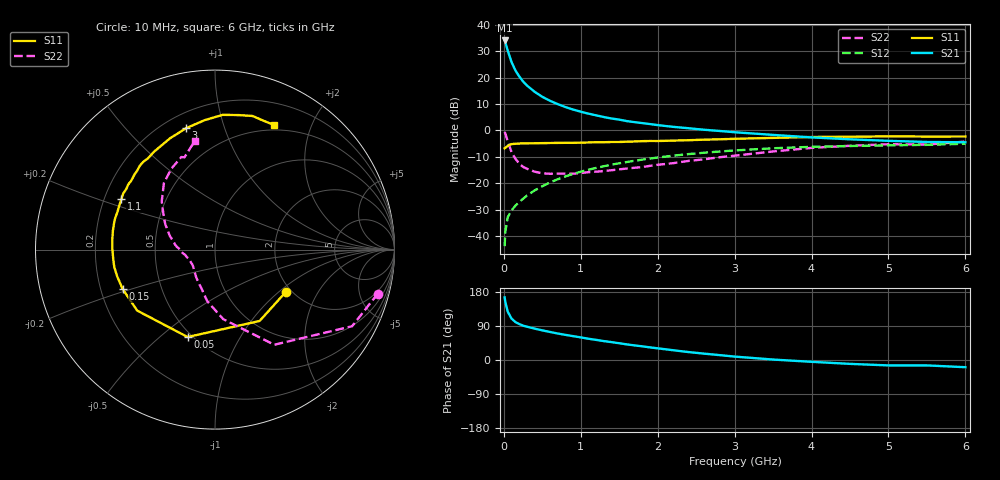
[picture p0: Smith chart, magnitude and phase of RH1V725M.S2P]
! SIEMENS Small Signal Semiconductors
! BFR106
! Si NPN RF Bipolar Junction Transistor in SOT23
! VCE = 1.75 V  IC = 25 mA
! Common Emitter S-Parameters:  August  1996
# GHz  S  MA  R  50
!  f  S11  S21  S12  S22
! GHz  MAG  ANG  MAG  ANG  MAG  ANG  MAG  ANG
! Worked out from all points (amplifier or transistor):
!   36 points, 10 MHz to 6 GHz, reference 50 ohm
!   highest |S21| = 34.1 dB at 10 MHz (marker M1)
!   |S21| within 3 dB of that: start of sweep to 42.11 MHz
!   unconditionally stable (mu >= 1): 317.8 MHz to 2.639 GHz; 5.017 GHz to end of sweep
!   at 250 MHz: K = 0.94, MSG = 22.2 dB, |S12| = -25.9 dB
!   at 1.4 GHz: K = 1.07, MAG = 7.1 dB, |S12| = -13.0 dB
!   at 6 GHz: K = 1.01, MAG = -0.4 dB, |S12| = -5.0 dB
!   S11 on the Smith chart (normalised r, x): 10 MHz: 1.87, -1.12; 50 MHz: 0.47, -0.62; 150 MHz: 0.29, -0.19; 1.1 GHz: 0.27, +0.23; 3 GHz: 0.29, +0.75; 6 GHz: 0.44, +1.49
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0.01  0.4597 -30.8  50.9 165.2  0.0064 80.8  0.94 -15.1
0.02  0.469 -58.0  46.89 153.0  0.0121 70.4  0.875 -29.2
0.05  0.5104 -107.4  32.8 127.8  0.0226 56.7  0.6245 -58.1
0.1  0.5508 -141.9  19.86 109.3  0.0305 52.0  0.3905 -83.2
0.15  0.5595 -156.9  13.79 100.2  0.0375 54.1  0.291 -98.5
0.2  0.565 -164.6  10.58 94.9  0.044 57.3  0.2353 -107.8
0.25  0.5695 -170.1  8.5 90.7  0.0507 60.0  0.2037 -117.1
0.3  0.5695 -174.3  7.132 87.8  0.0582 62.3  0.1878 -123.6
0.4  0.5723 179.2  5.414 82.8  0.0729 64.5  0.1656 -134.4
0.5  0.5751 174.1  4.346 78.2  0.0876 65.2  0.1541 -141.9
0.6  0.5783 169.7  3.652 74.0  0.1033 65.6  0.151 -146.8
0.7  0.5812 165.6  3.162 69.9  0.1189 65.4  0.1518 -151.6
0.9  0.5828 158.8  2.493 63.0  0.1501 63.8  0.1516 -159.6
1.1  0.5923 151.8  2.084 56.1  0.1801 61.7  0.1619 -164.7
1.3  0.5986 145.7  1.797 49.9  0.2101 58.9  0.1697 -170.3
1.6  0.613 137.2  1.505 41.2  0.2528 54.6  0.1896 -177.4
2.2  0.6426 121.8  1.172 25.8  0.3325 45.1  0.2397 168.1
3  0.6951 103.5  0.926 9.0  0.4182 32.1  0.3321 148.7
3.5  0.7234 94.6  0.824 1.2  0.46 24.4  0.4 137.9
4.5  0.761 80.0  0.68 -10.2  0.5068 9.8  0.5124 118.3
5.5  0.7669 68.8  0.605 -14.3  0.5338 0.9  0.5415 108.3
6  0.7685 64.8  0.597 -19.0  0.5594 -6.0  0.6152 100.6
